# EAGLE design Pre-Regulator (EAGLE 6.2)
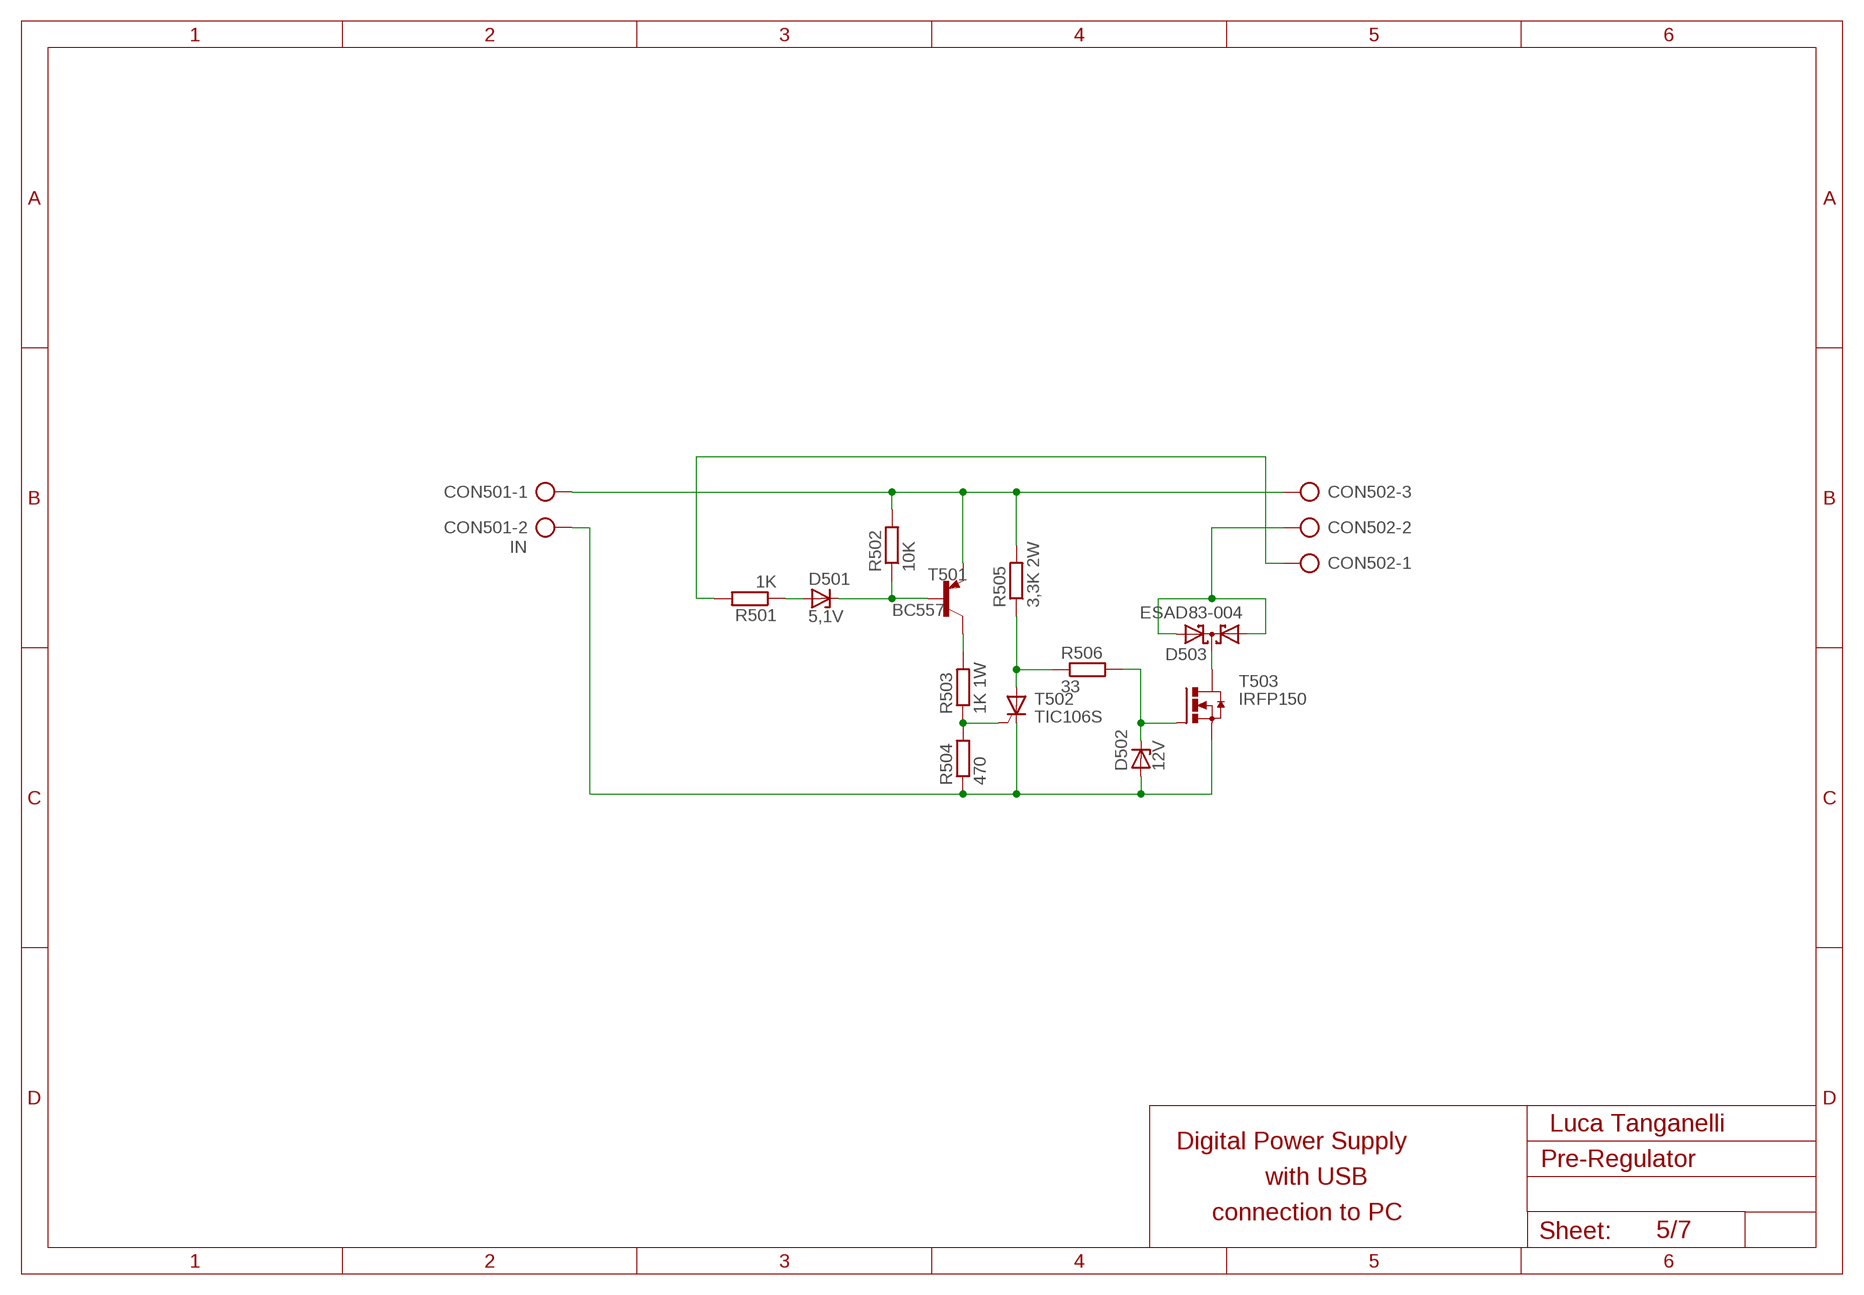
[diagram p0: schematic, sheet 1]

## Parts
CON501  IN  AK500/2  [AK500/2]
CON502  AK500/3  [AK500/3]
D501  5,1V  ZENER-DIODEDO35Z10  [DO35Z10]
D502  12V  ZENER-DIODEDO35Z10  [DO35Z10]
D503  ESAD83-004  ESAD83-004TO247BV  [TO247BV]
R501  1K  R-EU_0207/26  [0207/26]
R502  10K  R-EU_0207/10  [0207/10]
R503  1K 1W  R-EU_0921/26  [0921/26]
R504  470  R-EU_0207/10  [0207/10]
R505  3,3K 2W  R-EU_0921/26  [0921/26]
R506  33  R-EU_0207/10  [0207/10]
T501  BC557  BC557A-PNP-TO92-CBE  [TO92-CBE]
T502  TIC106S  [TIC106S]
T503  IRFP150  IRFP240  [TO247BV]

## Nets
N$1: CON501.1 CON502.3 R502.2 R505.P$2 T501.E
N$2: D503.C T503.C(D)
N$3: CON502.2 D503.B(A1) D503.E(A2)
N$4: CON501.2 D502.A R504.1 T502.C T503.E(S)
N$5: D502.C R506.2 T503.B(G)
N$6: R503.P$1 R504.2 T502.G
N$7: R505.P$1 R506.1 T502.A
N$8: R503.P$2 T501.C
N$9: D501.C R502.1 T501.B
N$10: D501.A R501.1
N$11: CON502.1 R501.2

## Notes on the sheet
- Luca Tanganelli
- Digital Power Supply
- with USB
- connection to PC
- 5/7

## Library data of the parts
CON501 = #-con-ptr500:AK500/2: CONNECTOR; OC_FARNELL: unknown; OC_NEWARK: unknown
CON502 = #-con-ptr500:AK500/3: CONNECTOR; OC_FARNELL: unknown; OC_NEWARK: unknown
D501 D502 = #-diode:ZENER-DIODE: Z-Diode
D503 = #-diode:ESAD83-004
R501-R506 = #-rcl:R-EU_: RESISTOR, European symbol
T501 = #-transistor:*-PNP-: PNP Transistror
T502 = triac:TIC106S: THYRISTOR
T503 = #-transistor-power:IRFP240: HEXFET Power MosFet Source: http://www.irf.com/

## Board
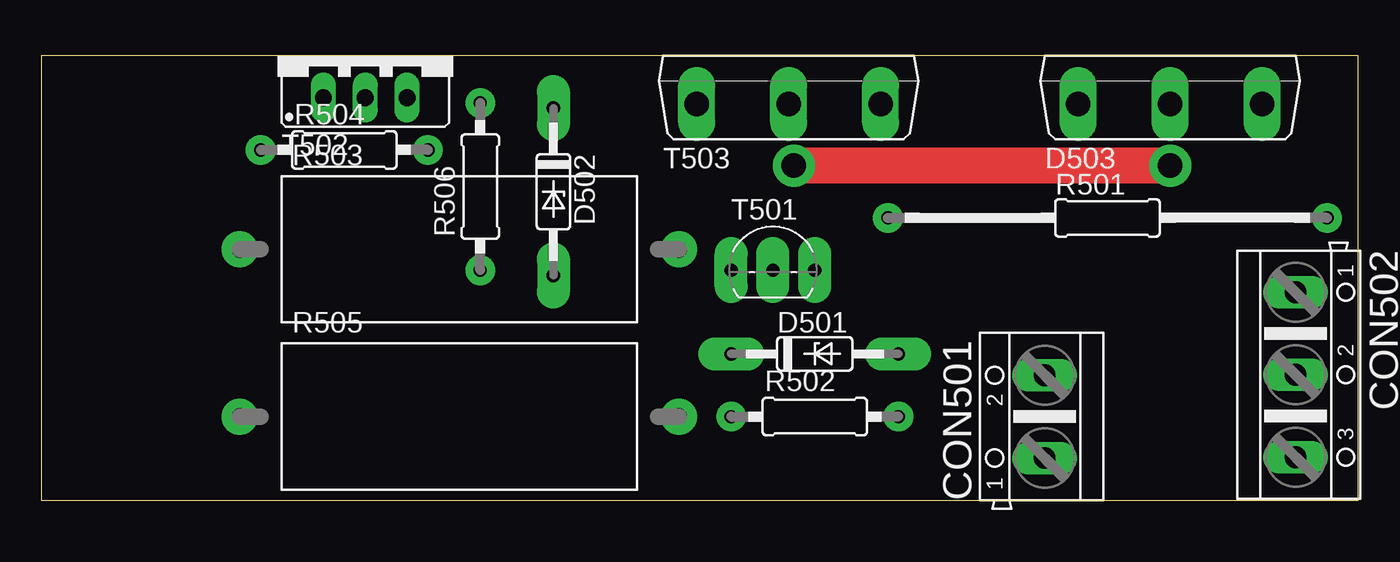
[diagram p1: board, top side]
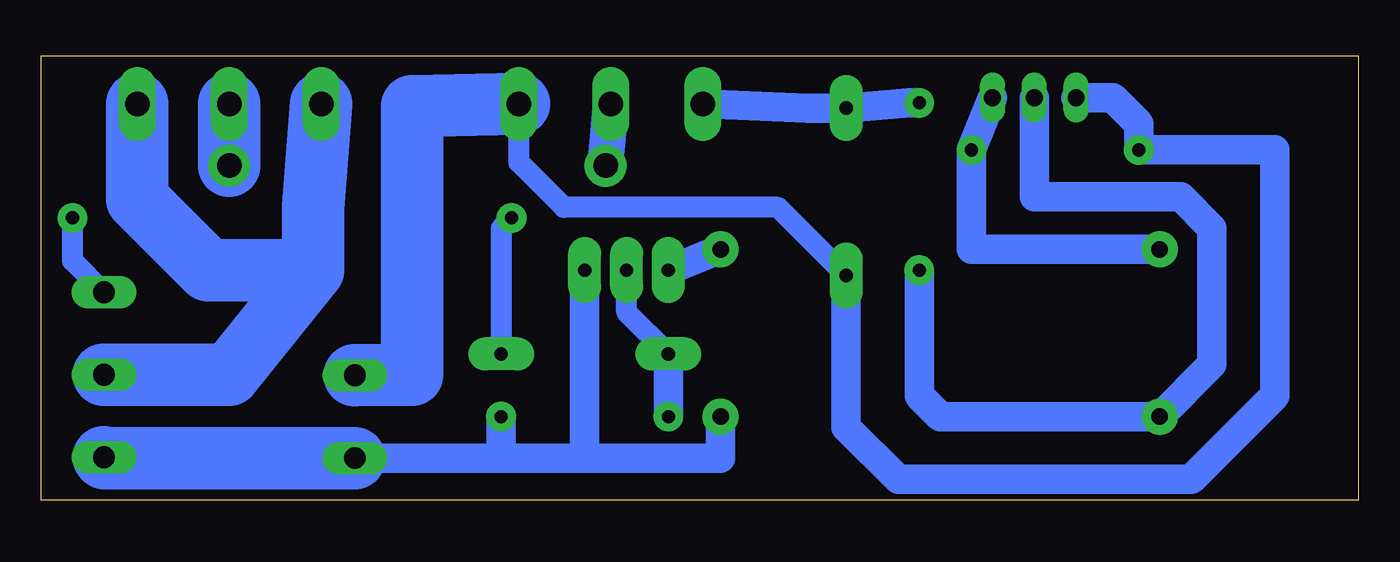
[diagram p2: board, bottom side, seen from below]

Size 80 x 27 mm. Coordinates in mm from the lower left corner, seen from the top.
Outline: 0,0 80,0 80,27 0,27 0,0
Copper layers (1*16): Top 0.035mm / dielectric 1.5mm / Bottom 0.035mm
Design rules: minimum track width 10mil, minimum drill 24mil, track to track 8mil, track to pad 8mil, pad to pad 8mil, via to via 8mil, smd to smd 8mil, copper to edge 40mil, drill to drill 8mil, minimum pad ring 10mil, minimum via ring 8mil, stop-mask expansion 4mil, vias tented up to drill 0mil, thermal gap 10mil

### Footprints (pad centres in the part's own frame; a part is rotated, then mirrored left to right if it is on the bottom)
AK500/2 = drill 1.321 pad 1.7 long: 1 -2.515,0; 2 2.515,0
AK500/3 = drill 1.321 pad 1.7 long: 1 -5.004,0; 2 0,0; 3 5.004,0
DO35Z10 = drill 0.813 pad 2 long: A 5.08,0; C -5.08,0
TO247BV = drill 1.499 pad 1.7 long: B -5.588,-2.921; C 0,-2.921; E 5.588,-2.921
0207/26 = drill 0.8 pad 1.8: 1 -13.335,0; 2 13.335,0
0207/10 = drill 0.8 pad 1.8: 1 -5.08,0; 2 5.08,0
0921/26 = drill 1 pad 2.184: P$1 -13.335,0; P$2 13.335,0
TO92-CBE = drill 0.813 pad 2 long: B 0,0; C -2.54,0; E 2.54,0
TIC106S = drill 1.016 long: A 0,-2.54; C -2.54,-2.54; G 2.54,-2.54

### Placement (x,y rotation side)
CON501  60.96,5.08 90 top
CON502  76.2,7.62 270 top
D501  46.99,8.89 0 top
D502  31.11,18.73 270 top
D503  68.58,26.99 0 top
R501  64.77,17.14 0 top
R502  46.99,5.08 0 top
R503  25.4,15.24 0 top
R504  18.41,21.27 0 top
R505  25.4,5.08 0 top
R506  26.67,19.05 90 top
T501  44.45,13.97 0 top
T502  19.68,26.99 0 top
T503  45.4,26.99 0 top

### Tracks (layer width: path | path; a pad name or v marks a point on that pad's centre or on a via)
N$1
  Bottom 1.778: R505.P$2 38.73,2.56 46.99,2.56 | 46.99,2.56 52.07,2.56 | 52.07,2.56 CON501.1 | T501.E 46.99,2.56 | R502.2 52.07,2.56
  Bottom 3.81: CON501.1 76.15,2.56 CON502.3
N$2  (via drill 1.5 pad 2.54)
  Top 2.184: v68.58,20.32 v45.72,20.32
  Bottom 2.184: v45.72,20.32 T503.C
  Bottom 3.81: D503.C v68.58,20.32
N$3
  Bottom 3.81: CON502.2 68.58,7.62 63.5,13.97 | 63.5,13.97 63.5,17.78 D503.B | D503.E 74.17,18.29 69.85,13.97 63.5,13.97
N$4
  Bottom 1.27: D502.A 35.24,17.78 48.26,17.78 50.99,20.51 T503.E
  Bottom 1.778: T502.C 14.92,24.45 13.34,22.86 R504.1 5.08,21.27 5.08,6.35 10.16,1.27 27.94,1.27 31.11,4.45 D502.A
  Bottom 3.81: CON501.2 58.42,7.62 57.47,7.62 57.47,23.94 T503.E
N$5
  Bottom 1.778: T503.B 33.47,23.81 D502.C 27.3,24.13 R506.2
N$6
  Bottom 1.778: R503.P$1 23.5,15.24 R504.2 T502.G
N$7
  Bottom 1.778: T502.A 19.68,18.41 10.79,18.41 8.89,16.51 8.89,8.26 R505.P$1 25.4,5.08 26.67,6.35 R506.1
N$8
  Bottom 1.778: T501.C R503.P$2
N$9
  Bottom 1.27: D501.C 44.45,11.43 T501.B
  Bottom 1.778: R502.1 D501.C
N$10
  Bottom 1.27: R501.1 52.07,16.51 D501.A
N$11
  Bottom 1.27: CON502.1 78.11,14.53 R501.2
